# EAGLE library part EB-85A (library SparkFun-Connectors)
EB-85A Connector Horizontal surface mount connector for the EB-85A/FV-M8 GPS receiver. Here is the connector we sell at SparkFun: Connector Horizontal SMD for EB-85A (GPS-08297) Datasheet It was also used on this SparkFun product: This connector is not on any currently live products, however it has been used on previously reitred products, so the package is proven.
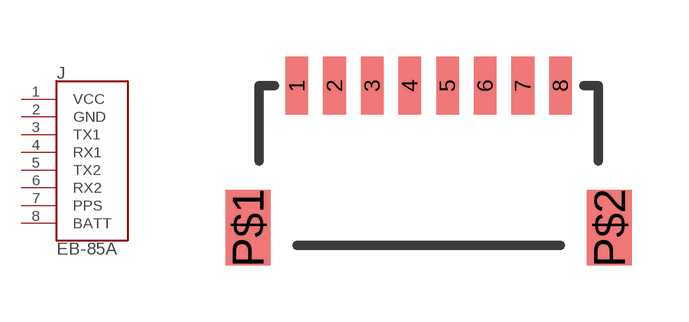
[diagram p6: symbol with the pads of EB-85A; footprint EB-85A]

Designator prefix J

## EB-85ASMD (PROD_ID: CONN-08435; SF_ID: GPS-08297)  [EB-85A]
1  VCC  pwr
2  GND  pwr
3  TX1  out
4  RX1  in
5  TX2  out
6  RX2  in
7  PPS  out
8  BATT  pwr

## Footprint EB-85A (pad centres in mm)
EB-85A Connector Horizontal surface mount connector for the EB-85A/FV-M8 GPS receiver. Specifications: Pin count: 10 Datasheet referenced for footprint Example device(s): EB-85A
smd 0.6 x 1.55: 1 0,0; 2 1,0; 3 2,0; 4 3,0; 5 4,0; 6 5,0; 7 6,0; 8 7,0
smd 1.2 x 2: P$1 -1.3,-3.775; P$2 8.3,-3.775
